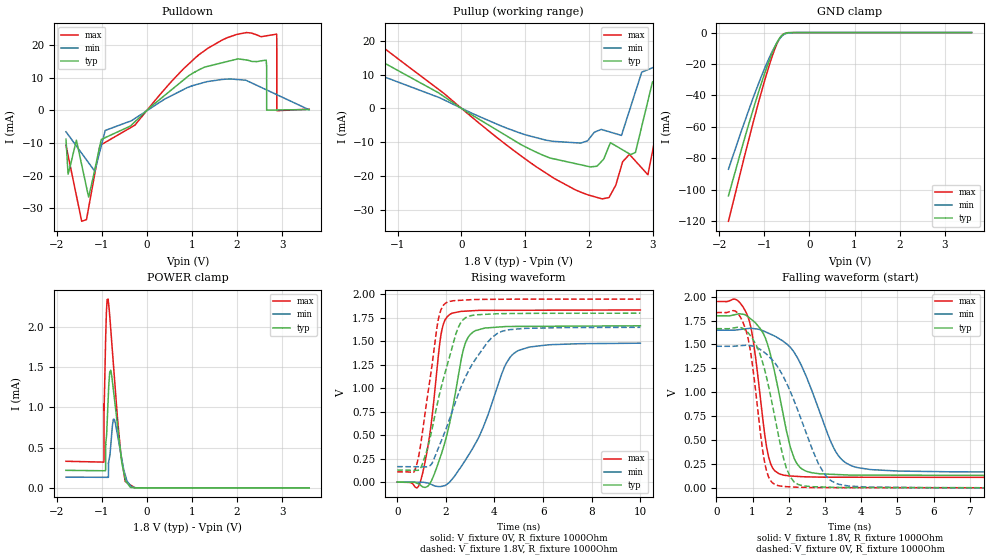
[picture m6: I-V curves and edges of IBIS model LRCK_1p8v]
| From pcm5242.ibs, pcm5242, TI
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|   Model
[Model]   LRCK_1p8v
Model_type   I/O
Polarity   Non-Inverting
Enable   Active-Low
Vinl = 0.54
Vinh = 1.26
Vmeas = 0.9
Vref = 0
Cref = 1pF
Rref = 1000000
|   typ   min   max
C_comp   1.346pF   1.304pF   1.384pF
[Voltage Range]   1.8   1.65   1.95
[Temperature Range]   27   105   -25
[Pullup Reference]   1.8   1.65   1.95
[Pulldown Reference]   -0   -0   -0
[Power Clamp Reference]   1.8   1.65   1.95
[GND Clamp Reference]   -0   -0   -0
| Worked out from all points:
|   slope of the pulldown table from 0 to 0.27 V, typ, clamps not added: 85.3 ohm
|   slope of the pullup table from 0 to 0.27 V, typ, clamps not added: 85.8 ohm
|   GND clamp passes 1 mA (typ) near -0.58 V on its own axis
|   POWER clamp passes 1 mA (typ) near -0.70 V on its own axis
|   falling waveform, V_fixture 1.8V, R_fixture 1000Ohm: 20-80 % time 577ps typ, 934ps min, 367ps max; typ from 1.8 V to 0.129 V
|   rising waveform, V_fixture 0V, R_fixture 1000Ohm: 20-80 % time 795ps typ, 1.39ns min, 491ps max; typ from 0 V to 1.67 V
|   rising waveform, V_fixture 1.8V, R_fixture 1000Ohm: 20-80 % time 946ps typ, 1.49ns min, 591ps max; typ from 0.129 V to 1.8 V
|   falling waveform, V_fixture 0V, R_fixture 1000Ohm: 20-80 % time 576ps typ, 948ps min, 364ps max; typ from 1.67 V to 0 V
[Pulldown]
|   Voltage   I(typ)   I(min)   I(max)
-1.8V     -8.858mA   -6.583mA   -10.72mA
-1.345V   -23.53mA   -15.18mA   -33.48mA
-1.047V   -10.86mA   -12.56mA   -10.79mA
2.21V     15.37mA    9.09mA     23.77mA
2.646V    15.32mA    6.278mA    22.77mA
2.657V    24.11uA    6.209mA    22.79mA
2.878V    69.33uA    4.786mA    23.3mA
2.882V    70.15uA    4.761mA    21.6mA
2.882V    70.17uA    4.76mA     19.04mA
2.882V    70.18uA    4.76mA     2.875mA
2.882V    70.19uA    4.759mA    -145.8uA
3.6V      217.2uA    134uA      327uA
[GND Clamp]
|   Voltage   I(typ)   I(min)   I(max)
-1.8V     -103.9mA   -86.97mA   -120.1mA
-1.529V   -76.2mA    -63.93mA   -88.66mA
-1.366V   -59.98mA   -50.79mA   -70.14mA
-1.129V   -37.66mA   -32.31mA   -44.12mA
-982.5mV  -24.93mA   -21.81mA   -29.21mA
-885.8mV  -17.25mA   -15.56mA   -20.11mA
-751.8mV  -8.033mA   -7.956mA   -9.149mA
-654.8mV  -3.201mA   -3.678mA   -3.345mA
-581.1mV  -1.127mA   -1.505mA   -929.5uA
-519.1mV  -391.7uA   -538.9uA   -381.2uA
-344.1mV  -2.999uA   -11.08uA   -25.67uA
3.6V      0A         0A         0A
[Pullup]
|   Voltage   I(typ)   I(min)   I(max)
-1.8V     4.586mA    915uA      12.69mA
-1.762V   4.781mA    1.64mA     23.04mA
-1.487V   16.25mA    6.868mA    21.63mA
2.21V     -15.46mA   -6.296mA   -26.75mA
2.732V    -13.03mA   4.904mA    -15.56mA
2.928V    2.196mA    11.45mA    -19.62mA
3.152V    9.141mA    13.17mA    1.967mA
3.38V     11.08mA    14.91mA    4.1mA
3.4V      11.25mA    -4.945mA   4.285mA
3.421V    -12.48mA   -25.9mA    4.48mA
3.49V     -91.24mA   -95.44mA   -82.36mA
3.6V      -112.5mA   -105.5mA   -117.8mA
[POWER Clamp]
|   Voltage   I(typ)   I(min)   I(max)
-1.8V     217.2uA    133.2uA    329.4uA
-957.7mV  212uA      130.7uA    319.3uA
-955.2mV  211.9uA    130.7uA    347.5uA
-955.2mV  211.9uA    130.7uA    447.8uA
-955.1mV  211.9uA    130.7uA    1.04mA
-922mV    211.7uA    130.6uA    1.771mA
-917.8mV  547.1uA    130.6uA    1.88mA
-864.8mV  1.078mA    130.5uA    2.34mA
-828.4mV  1.435mA    393.8uA    2.132mA
-747.2mV  1.215mA    850.8uA    1.536mA
-484.3mV  107.9uA    160.8uA    78.57uA
3.6V      0A         0A         0A
[Ramp]
R_load = 1000
|   typ   min   max
dV/dt_r   0.999416/7.94516e-10   0.888237/1.38677e-09   1.10076/4.90449e-10
dV/dt_f   1.00287/5.76676e-10   0.891028/9.33072e-10   1.10474/3.6742e-10
[Falling Waveform]
V_fixture = 1.8V
V_fixture_min = 1.65V
V_fixture_max = 1.95V
R_fixture = 1000Ohm
C_fixture = 0F
|   Time   V(typ)   V(min)   V(max)
0s        1.8V       1.65V      1.95V
878.8ps   1.79V      1.667V     1.785V
1.041ns   1.74V      1.666V     1.484V
1.393ns   1.527V     1.626V     417mV
1.724ns   1.004V     1.563V     149.8mV
2.045ns   424.5mV    1.47V      124.4mV
2.302ns   217.8mV    1.316V     118.2mV
3.252ns   140.6mV    409mV      111.5mV
3.733ns   133.8mV    230.8mV    111.3mV
10ns      128.6mV    165mV      108.8mV
[Rising Waveform]
V_fixture = 0V
V_fixture_min = 0V
V_fixture_max = 0V
R_fixture = 1000Ohm
C_fixture = 0F
|   Time   V(typ)   V(min)   V(max)
0s        1.409nV    53.34nV    589.8pV
956.1ps   -31.89mV   -1.566mV   5.969mV
1.341ns   -16.74mV   -17.7mV    509.7mV
1.809ns   294.1mV    -46.04mV   1.583V
2.166ns   641.2mV    3.134mV    1.788V
2.673ns   1.358V     181.7mV    1.82V
2.919ns   1.544V     281.4mV    1.824V
4.402ns   1.657V     1.222V     1.831V
4.782ns   1.659V     1.368V     1.831V
10ns      1.666V     1.48V      1.835V
[Rising Waveform]
V_fixture = 1.8V
V_fixture_min = 1.65V
V_fixture_max = 1.95V
R_fixture = 1000Ohm
C_fixture = 0F
|   Time   V(typ)   V(min)   V(max)
0s        128.5mV    164.8mV    108.8mV
654.1ps   126.3mV    163.8mV    102.8mV
798.8ps   125.8mV    163.5mV    184.5mV
1.207ns   327.7mV    163.1mV    848.3mV
1.668ns   854.6mV    346.9mV    1.703V
1.982ns   1.178V     550.9mV    1.905V
2.422ns   1.586V     872.4mV    1.935V
2.698ns   1.727V     1.057V     1.939V
4.148ns   1.795V     1.588V     1.948V
10ns      1.8V       1.65V      1.95V
[Falling Waveform]
|Gnd
V_fixture = 0V
V_fixture_min = 0V
V_fixture_max = 0V
R_fixture = 1000Ohm
C_fixture = 0F
|   Time   V(typ)   V(min)   V(max)
0s        1.666V     1.482V     1.835V
798.8ps   1.65V      1.492V     1.67V
956.1ps   1.585V     1.487V     1.397V
1.341ns   1.227V     1.413V     252.1mV
1.62ns    732.3mV    1.305V     34.62mV
1.936ns   204.5mV    1.098V     12.7mV
2.153ns   60.35mV    906.4mV    7.915mV
2.822ns   10.3mV     249.9mV    2.681mV
3.302ns   5.115mV    47.66mV    2.502mV
10ns      5.968uV    98.2uV     2.238uV
